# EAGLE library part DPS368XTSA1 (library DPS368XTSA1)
Infineon PRESSURE SENSOR Source: Datasheet
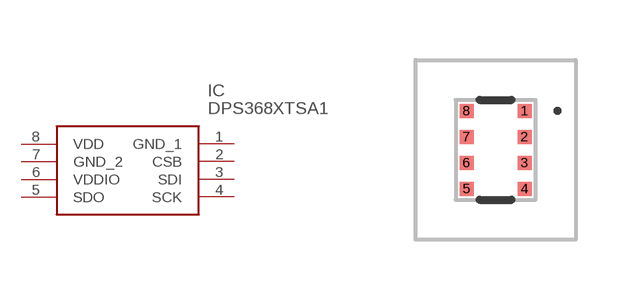
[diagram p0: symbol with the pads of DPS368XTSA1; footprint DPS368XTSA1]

Designator prefix IC

## DPS368XTSA1 (Description: Infineon PRESSURE SENSOR; Height: 1.1mm; Manufacturer_Name: Infineon; Manufacturer_Part_Number: DPS368XTSA1; Mouser_Part_Number: 726-DPS368XTSA1; Mouser_Price-Stock: https://www.mouser.co.uk/ProductDetail/Infineon-Technologies/DPS368XTSA1?qs=l7cgNqFNU1issZx9oeCNag%3D%3D)  [DPS368XTSA1]
1  GND_1
2  CSB
3  SDI
4  SCK
5  SDO
6  VDDIO
7  GND_2
8  VDD

## Footprint DPS368XTSA1 (pad centres in mm)
DPS368XTSA1-4
smd 0.35 x 0.35: 1 0.725,0.975; 2 0.725,0.325; 3 0.725,-0.325; 4 0.725,-0.975; 5 -0.725,-0.975; 6 -0.725,-0.325; 7 -0.725,0.325; 8 -0.725,0.975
